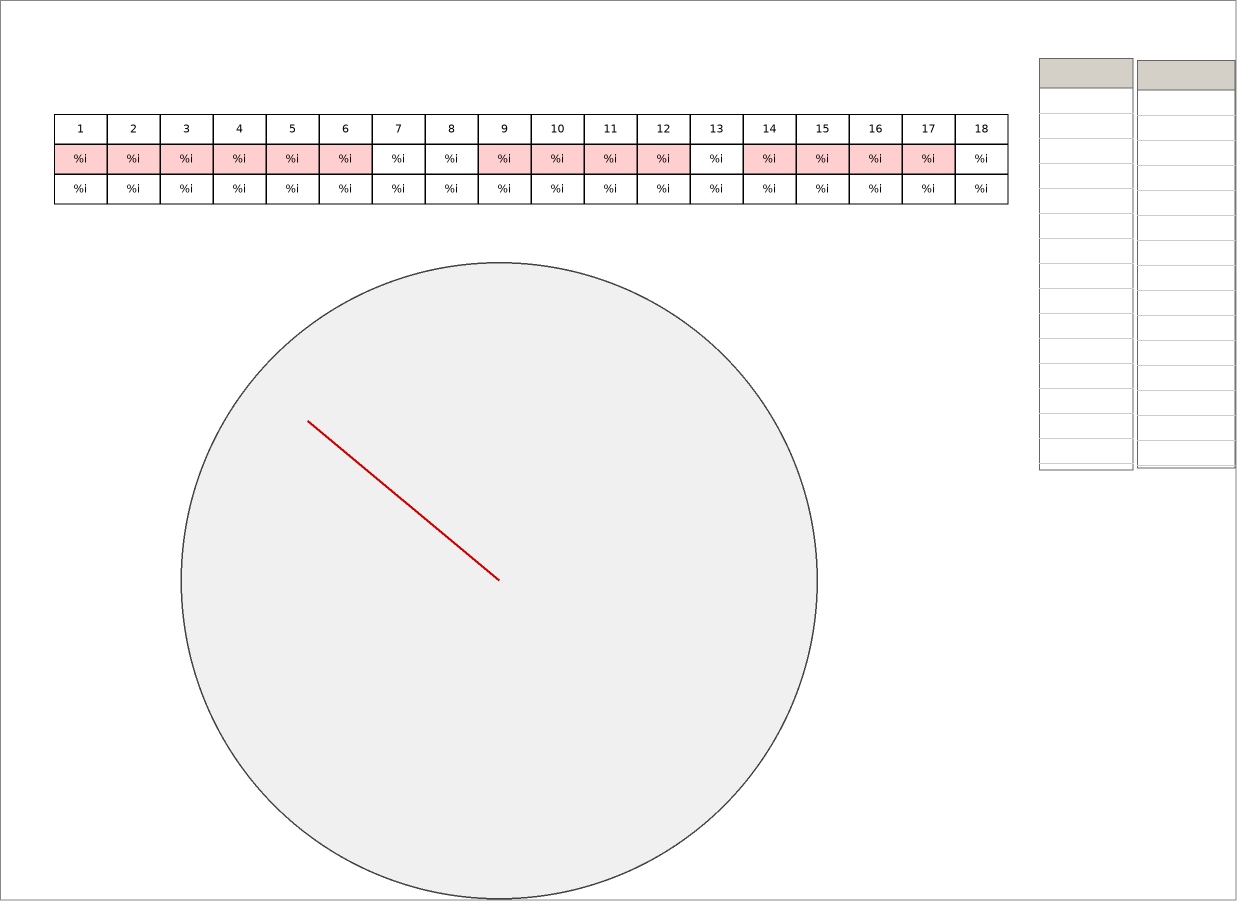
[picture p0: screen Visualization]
VISUALIZATION Visualization  // 1237x901
    Rectangle (54,114 53x30), "1"
    Rectangle (54,144 53x30), "%i", text variable: MAIN.bStartSerialData[1]
    Rectangle (54,174 53x30), "%i", text variable: MAIN.bSerialData[1]
    Rectangle (107,114 53x30), "2"
    Rectangle (107,144 53x30), "%i", text variable: MAIN.bStartSerialData[2]
    Rectangle (107,174 53x30), "%i", text variable: MAIN.bSerialData[2]
    Rectangle (160,114 53x30), "3"
    Rectangle (160,144 53x30), "%i", text variable: MAIN.bStartSerialData[3]
    Rectangle (160,174 53x30), "%i", text variable: MAIN.bSerialData[3]
    Rectangle (213,114 53x30), "4"
    Rectangle (213,144 53x30), "%i", text variable: MAIN.bStartSerialData[4]
    Rectangle (213,174 53x30), "%i", text variable: MAIN.bSerialData[4]
    Rectangle (266,114 53x30), "5"
    Rectangle (266,144 53x30), "%i", text variable: MAIN.bStartSerialData[5]
    Rectangle (266,174 53x30), "%i", text variable: MAIN.bSerialData[5]
    Rectangle (319,114 53x30), "6"
    Rectangle (319,144 53x30), "%i", text variable: MAIN.bStartSerialData[6]
    Rectangle (319,174 53x30), "%i", text variable: MAIN.bSerialData[6]
    Rectangle (372,114 53x30), "7"
    Rectangle (372,144 53x30), "%i", text variable: MAIN.bStartSerialData[7]
    Rectangle (372,174 53x30), "%i", text variable: MAIN.bSerialData[7]
    Rectangle (425,114 53x30), "8"
    Rectangle (425,144 53x30), "%i", text variable: MAIN.bStartSerialData[8]
    Rectangle (425,174 53x30), "%i", text variable: MAIN.bSerialData[8]
    Rectangle (478,114 53x30), "9"
    Rectangle (478,144 53x30), "%i", text variable: MAIN.bStartSerialData[9]
    Rectangle (478,174 53x30), "%i", text variable: MAIN.bSerialData[9]
    Rectangle (531,114 53x30), "10"
    Rectangle (531,144 53x30), "%i", text variable: MAIN.bStartSerialData[10]
    Rectangle (531,174 53x30), "%i", text variable: MAIN.bSerialData[10]
    Rectangle (584,114 53x30), "11"
    Rectangle (584,144 53x30), "%i", text variable: MAIN.bStartSerialData[11]
    Rectangle (584,174 53x30), "%i", text variable: MAIN.bSerialData[11]
    Rectangle (637,114 53x30), "12"
    Rectangle (637,144 53x30), "%i", text variable: MAIN.bStartSerialData[12]
    Rectangle (637,174 53x30), "%i", text variable: MAIN.bSerialData[12]
    Rectangle (690,114 53x30), "13"
    Rectangle (690,144 53x30), "%i", text variable: MAIN.bStartSerialData[13]
    Rectangle (690,174 53x30), "%i", text variable: MAIN.bSerialData[13]
    Rectangle (743,114 53x30), "14"
    Rectangle (743,144 53x30), "%i", text variable: MAIN.bStartSerialData[14]
    Rectangle (743,174 53x30), "%i", text variable: MAIN.bSerialData[14]
    Rectangle (796,114 53x30), "15"
    Rectangle (796,144 53x30), "%i", text variable: MAIN.bStartSerialData[15]
    Rectangle (796,174 53x30), "%i", text variable: MAIN.bSerialData[15]
    Rectangle (849,114 53x30), "16"
    Rectangle (849,144 53x30), "%i", text variable: MAIN.bStartSerialData[16]
    Rectangle (849,174 53x30), "%i", text variable: MAIN.bSerialData[16]
    Rectangle (902,114 53x30), "17"
    Rectangle (902,144 53x30), "%i", text variable: MAIN.bStartSerialData[17]
    Rectangle (902,174 53x30), "%i", text variable: MAIN.bSerialData[17]
    Rectangle (955,114 53x30), "18"
    Rectangle (955,144 53x30), "%i", text variable: MAIN.bStartSerialData[18]
    Rectangle (955,174 53x30), "%i", text variable: MAIN.bSerialData[18]
    Table (1039,58 94x412), data array: MAIN.fbSentDecode.nSlowChnBufferB2
        p3854506369: MAIN.fbSentDecode.nSlowChnBufferB2[INDEX]
    Table (1137,60 98x408), data array: MAIN.fbSentDecode.nSlowChnBufferB3
        p3854506369: MAIN.fbSentDecode.nSlowChnBufferB3[INDEX]
    Meter360 (88,262 822x637), value: MAIN.fFastDataPresureCh2, style: Meter-Meter360-Gray, scale format: %.1f, scale 0..5
END_VISUALIZATION
